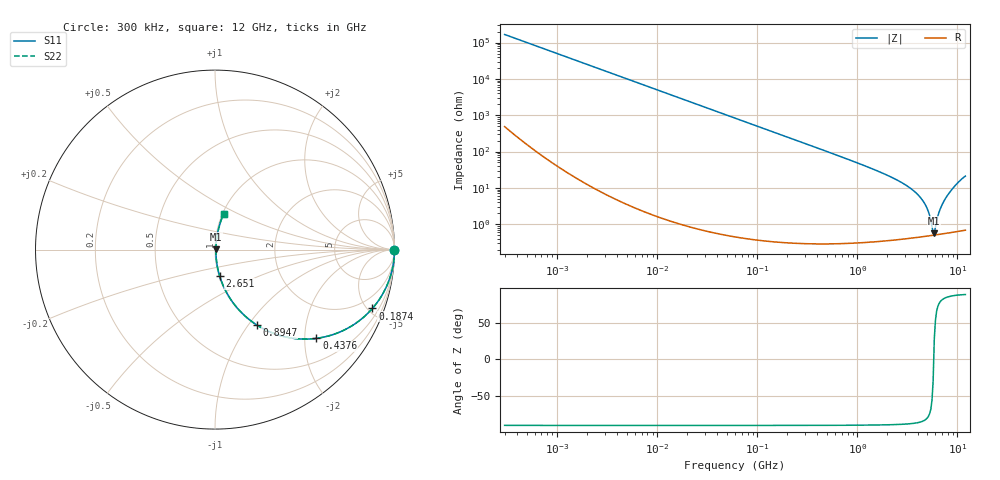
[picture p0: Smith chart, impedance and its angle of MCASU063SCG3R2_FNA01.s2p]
! MCASU063SCG3R2_FNA01  S-PARAMETER MODEL  ( General Type )
! Model Generated by TAIYO YUDEN Corporation (http://www.ty-top.com)
! Version 1.0
! TAIYO YUDEN Control No. 130801
! Copyright(c) 2013 TAIYO YUDEN CO.,LTD. All Rights Reserved.
! Product Description (link to TY-COMPAS)
! https://ds.yuden.co.jp/TYCOMPAS/or/detail?pn=MCASU063SCG3R2CFNA01&u=M
! Products Name : Multilayer Ceramic Capacitors
! Characteristics :
!  Capacitance : 3.2 pF , Rated Voltage : 50V , TCC : CG / C0G
!  Case Size : 0.6 x 0.3 / 0.024 x 0.012 [mm/inch] , Thickness : 0.3 / 0.012 [mm/inch]
!  (Conditions: Temperature = 25 degC , DC Bias Current/Voltage = 0A / 0V)
! External Node Assignments :
!  1  o---| |---o  2
! GND o---------o GND
! Frequency Range : 0.3MHz  -  12000MHz  [ 401 STEP ]
# MHz S RI R 50
! Freq[MHz].  S11 Real  S11 Imag  S21 Real  S21 Imag  S12 Real  S12 Imag  S22 Real  S22 Imag
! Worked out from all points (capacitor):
!   401 points, 300 kHz to 12 GHz, reference 50 ohm
!   read as one part in series: C = 3.17 pF near 316.3 kHz
!   lowest |Z| = 564 mohm at 5.869 GHz (marker M1)
!   series resonance near 5.795 GHz, so ESL is about 240 pH
!   S11 on the Smith chart (normalised r, x): 300 kHz: open; 187.4 MHz: 1.01, -5.35; 437.6 MHz: 1.01, -2.28; 894.7 MHz: 1.01, -1.10; 2.651 GHz: 1.01, -0.30; 12 GHz: 1.01, +0.42
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0.3  1 -0.000598  2.09e-06 0.000598  2.09e-06 0.000598  1 -0.000598
1.769972  1 -0.00353  1.43e-05 0.00353  1.43e-05 0.00353  1 -0.00353
10.44266  0.9996 -0.0208  0.00044 0.0208  0.00044 0.0208  0.9996 -0.0208
60  0.9858 -0.1179  0.0142 0.1179  0.0142 0.1179  0.9858 -0.1179
187.4445  0.8771 -0.3278  0.1229 0.3278  0.1229 0.3278  0.8771 -0.3278
353.9943  0.6658 -0.4707  0.3342 0.4707  0.3342 0.4707  0.6658 -0.4707
437.5599  0.5651 -0.4945  0.4349 0.4945  0.4349 0.4945  0.5651 -0.4945
894.6982  0.2319 -0.4193  0.7681 0.4193  0.7681 0.4193  0.2319 -0.4193
1331.232  0.1153 -0.315  0.8847 0.315  0.8847 0.315  0.1153 -0.315
2088.533  0.045 -0.1991  0.955 0.1991  0.955 0.1991  0.045 -0.1991
2650.866  0.0255 -0.1455  0.9745 0.1455  0.9745 0.1455  0.0255 -0.1455
3547.679  0.0118 -0.0872  0.9882 0.0872  0.9882 0.0872  0.0118 -0.0872
4385.161  0.00683 -0.0486  0.9932 0.0486  0.9932 0.0486  0.00683 -0.0486
5006.236  0.00533 -0.0254  0.9947 0.0254  0.9947 0.0254  0.00533 -0.0254
5565.855  0.00493 -0.00719  0.9951 0.00719  0.9951 0.00719  0.00493 -0.00719
5715.274  0.00493 -0.00276  0.9951 0.00276  0.9951 0.00276  0.00493 -0.00276
5868.704  0.00498 0.00257  0.995 -0.00257  0.995 -0.00257  0.00498 0.00257
6026.253  0.00507 0.00669  0.9949 -0.00669  0.9949 -0.00669  0.00507 0.00669
6699.894  0.00586 0.0247  0.9941 -0.0247  0.9941 -0.0247  0.00586 0.0247
7648.807  0.00827 0.0519  0.9917 -0.0519  0.9917 -0.0519  0.00827 0.0519
9708.23  0.021 0.1204  0.979 -0.1204  0.979 -0.1204  0.021 0.1204
12000  0.0485 0.1991  0.9515 -0.1991  0.9515 -0.1991  0.0485 0.1991
